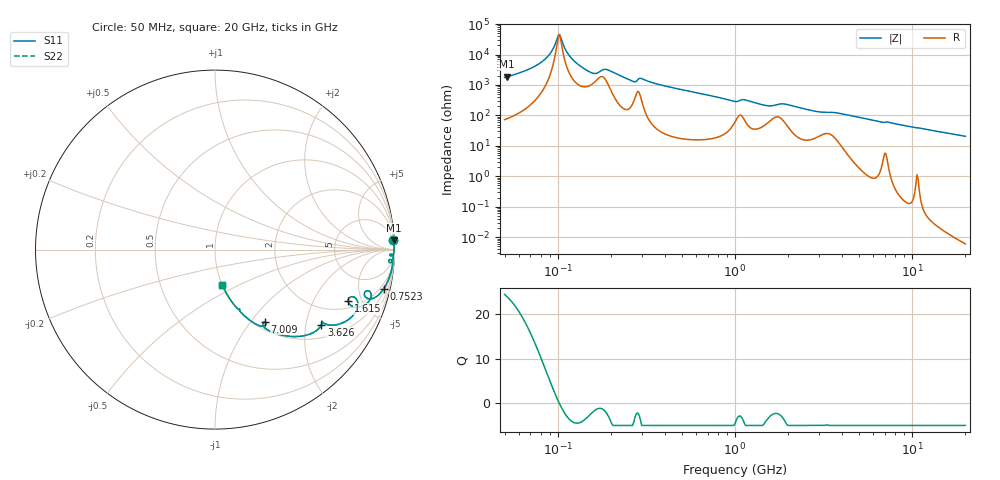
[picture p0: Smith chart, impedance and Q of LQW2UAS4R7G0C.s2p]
!Murata Part Number: LQW2UAS4R7G0C
!These Parameters are Measured in Series Mode Connection
!  o--[Z]--o
!Port1  Port2
!  o-------o
!Freq. Start=50[MHz] Stop=20[GHz], 401[Steps]
# Hz S RI R 50
!Freq.(Hz) S11(Real) S11(Imag) S21(Real) S21(Imag) S12(Real) S12(Imag) S22(Real) S22(Imag)
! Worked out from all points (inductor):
!   401 points, 50 MHz to 20 GHz, reference 50 ohm
!   read as one part in series: L = 4.22 uH near 51.52 MHz
!   highest Q = 23.9 at 51.52 MHz (marker M1), where L = 5.71 uH
!   self-resonance near 101.1 MHz
!   S11 on the Smith chart (normalised r, x): 50 MHz: 2, +35; 752.3 MHz: 1.35, -8.52; 1.615 GHz: 2.47, -3.86; 3.626 GHz: 1.38, -2.45; 7.009 GHz: 1.11, -1.17; 20 GHz: 1.00, -0.41
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5e7  0.9945 0.0562  0.0055 -0.0562  0.0055 -0.0562  0.9945 0.0562
5.152053e7  0.9949 0.0536  0.00514 -0.0536  0.00514 -0.0536  0.9949 0.0536
8.196717e7  0.9979 0.0164  0.00206 -0.0164  0.00206 -0.0164  0.9979 0.0164
9.102821e7  0.998 0.00852  0.00196 -0.00852  0.00196 -0.00852  0.998 0.00852
1.010909e8  0.9979 0.000516  0.00213 -0.000516  0.00213 -0.000516  0.9979 0.000516
1.041651e8  0.9978 -0.00181  0.00224 0.00181  0.00224 0.00181  0.9978 -0.00181
1.1568e8  0.997 -0.0102  0.00298 0.0102  0.00298 0.0102  0.997 -0.0102
1.364002e8  0.9933 -0.0249  0.00666 0.0249  0.00666 0.0249  0.9933 -0.0249
1.584406e8  0.9796 -0.0352  0.0204 0.0352  0.0204 0.0352  0.9796 -0.0352
1.868199e8  0.986 -0.027  0.014 0.027  0.014 0.027  0.986 -0.027
2.636584e8  0.9817 -0.0718  0.0183 0.0718  0.0183 0.0718  0.9817 -0.0718
2.972233e8  0.985 -0.0592  0.015 0.0592  0.015 0.0592  0.985 -0.0592
3.721004e8  0.9879 -0.0952  0.0121 0.0952  0.0121 0.0952  0.9879 -0.0952
7.523192e8  0.9398 -0.2182  0.0602 0.2182  0.0602 0.2182  0.9398 -0.2182
1e9  0.8445 -0.2693  0.1555 0.2693  0.1555 0.2693  0.8445 -0.2693
1.614971e9  0.7424 -0.2863  0.2576 0.2863  0.2576 0.2863  0.7424 -0.2863
2.021818e9  0.7915 -0.3296  0.2085 0.3296  0.2085 0.3296  0.7915 -0.3296
2.728004e9  0.6553 -0.4211  0.3447 0.4211  0.3447 0.4211  0.6553 -0.4211
3.626126e9  0.5924 -0.4191  0.4076 0.4191  0.4076 0.4191  0.5924 -0.4191
7.009217e9  0.2768 -0.4014  0.7232 0.4014  0.7232 0.4014  0.2768 -0.4014
7.442007e9  0.26 -0.4265  0.74 0.4265  0.74 0.4265  0.26 -0.4265
2e10  0.0407 -0.1975  0.9593 0.1975  0.9593 0.1975  0.0407 -0.1975
